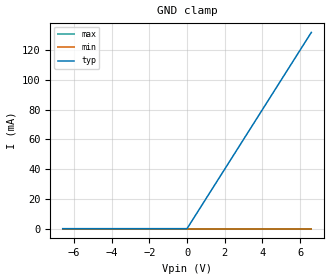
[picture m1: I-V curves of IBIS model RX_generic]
[IBIS Ver]   5.0
[File Name]   RX_generic.ibs
[File Rev]   1.0
[Component]   RX_generic
[Manufacturer] My Company
[Package]
R_pkg  0.0   NA   NA
L_pkg  0.0   NA   NA
C_pkg  0.0   NA   NA
[Pin]   signal_name   model_name   R_pin L_pin  C_pin
2p   RX_generic_2p   RX_generic
2n   RX_generic_2n   RX_generic
[Diff_Pin] inv_pin vdiff tdelay_typ tdelay_min tdelay_max
2p   2n   NA   NA   NA   NA
| Models and submodels in the file (1): RX_generic (Input)
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[Model] RX_generic
Model_type Input
C_comp 0p 0p 0p
Vinh = 0.25
Vinl = -0.25
[Temperature_Range] 25 125 0
[Voltage Range] 1.0 1.0 1.0
[Algorithmic Model]
Executable Windows_cl16.00.30319.01_64 RX_generic_x64.dll RX_generic.ami
Executable Windows_cl16.00.30319.01_32 RX_generic.dll RX_generic.ami
[End Algorithmic Model]
[GND Clamp]
-6.6V     0A         0A         0A
0V        0A         0A         0A
6.6V      132mA      0A         0A
[Power Clamp]
-6.6V     0A         0A         0A
0V        0A         0A         0A
6.6V      0A         0A         0A
